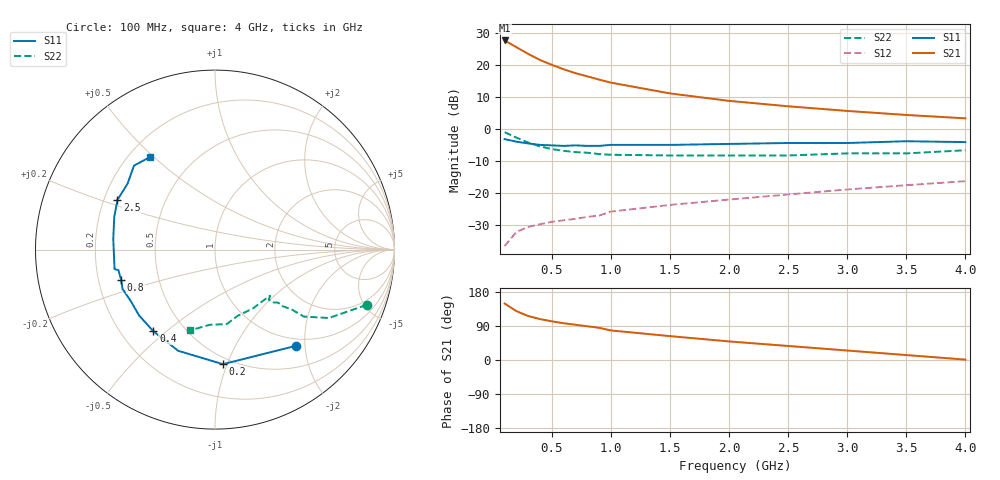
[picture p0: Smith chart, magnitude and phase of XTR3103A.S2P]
! HXTR-3103  (2N6838) Common Emitter
! Vce=10V  Ic=10mA
# ghz s ma r 50
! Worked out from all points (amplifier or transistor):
!   16 points, 100 MHz to 4 GHz, reference 50 ohm
!   highest |S21| = 27.7 dB at 100 MHz (marker M1)
!   |S21| within 3 dB of that: start of sweep to 242.9 MHz
!   unconditionally stable (mu >= 1): 896.6 MHz to 907.6 MHz; 1.133 GHz to 3.099 GHz
!   at 300 MHz: K = 0.44, MSG = 27.0 dB, |S12| = -30.5 dB
!   at 900 MHz: K = 1.00, MAG = 20.9 dB, |S12| = -26.9 dB
!   at 4 GHz: K = 0.86, MSG = 9.8 dB, |S12| = -16.2 dB
!   S11 on the Smith chart (normalised r, x): 100 MHz: 0.86, -1.82; 200 MHz: 0.45, -0.97; 400 MHz: 0.34, -0.45; 800 MHz: 0.30, -0.14; 2.5 GHz: 0.26, +0.23; 4 GHz: 0.28, +0.49
0.1  0.7 -50.0  24.26 149.0  0.015 60.0  0.9 -20.0
0.2  0.64 -86.0  19.05 129.0  0.025 49.0  0.74 -31.0
0.3  0.6 -110.0  14.96 116.0  0.03 43.0  0.62 -37.0
0.4  0.57 -127.0  12.02 108.0  0.033 41.0  0.54 -38.0
0.5  0.56 -139.0  10.11 102.0  0.036 41.0  0.49 -40.0
0.6  0.55 -149.0  8.61 97.0  0.038 42.0  0.46 -40.0
0.7  0.56 -157.0  7.49 93.0  0.04 43.0  0.44 -42.0
0.8  0.55 -162.0  6.68 89.0  0.043 44.0  0.43 -42.0
0.9  0.55 -168.0  5.95 85.0  0.045 46.0  0.41 -43.0
1  0.57 -169.0  5.33 78.0  0.052 42.0  0.4 -40.0
1.5  0.57 174.0  3.62 63.0  0.066 48.0  0.39 -48.0
2  0.59 162.0  2.77 49.0  0.08 48.0  0.39 -57.0
2.5  0.61 153.0  2.28 37.0  0.096 48.0  0.39 -71.0
3  0.61 143.0  1.93 25.0  0.115 45.0  0.42 -81.0
3.5  0.65 134.0  1.67 13.0  0.134 43.0  0.42 -94.0
4  0.63 125.0  1.48 1.0  0.155 39.0  0.47 -107.0
